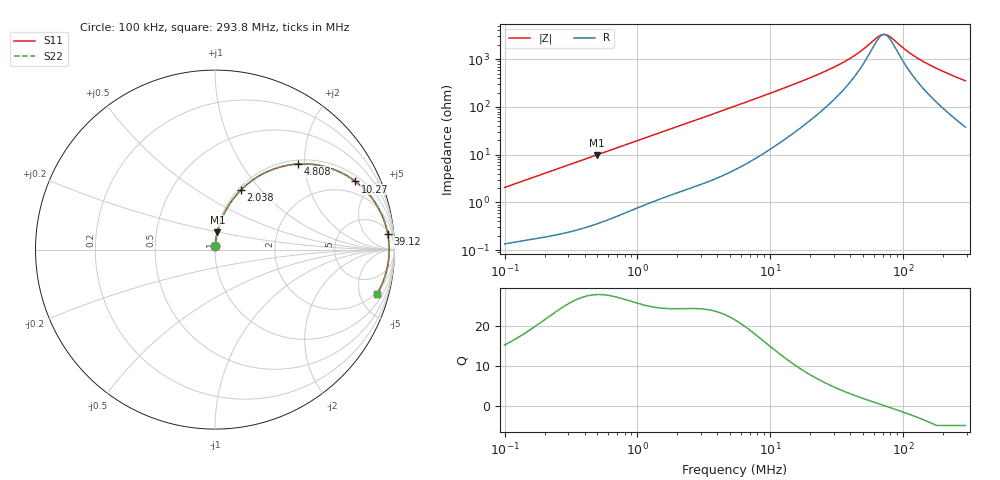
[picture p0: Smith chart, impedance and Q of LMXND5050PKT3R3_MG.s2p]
! LMXND5050PKT3R3_MG  S-PARAMETER MODEL  ( General Type )
! Model Generated by TAIYO YUDEN Corporation (http://www.ty-top.com)
! Version 1.0
! TAIYO YUDEN Control No. 191023NI43SB-FBB
! Copyright(c) 2019 TAIYO YUDEN CO.,LTD. All Rights Reserved.
! Product Description (link to TY-COMPAS)
! https://ds.yuden.co.jp/TYCOMPAS/or/detail?pn=LMXND5050PKT3R3NMG&u=M
! Products Name : Inductors
! Characteristics :
!  Inductance : 3.3 uH , SRF(min) : 48 MHz , DC Resistance(max) : 0.096 Ohm
!  Rated Current : Saturation :2350 mA , Temp Rise : 1700 mA
!  Case Size : 4.9 x 4.9 / 0.193 x 0.193 [mm/inch] , Thickness : 1.4 / 0.055 [mm/inch]
!  (Conditions: Temperature = 25 degC , DC Bias Current/Voltage = 0A / 0V)
! External Node Assignments :
!  1  o---GGG---o  2
! GND o---------o GND
! Frequency Range : 0.1MHz  -  293.796821MHz  [ 402 STEP ]
# MHz S RI R 50
! Freq[MHz].  S11 Real  S11 Imag  S21 Real  S21 Imag  S12 Real  S12 Imag  S22 Real  S22 Imag
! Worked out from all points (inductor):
!   401 points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, 100 kHz to 293.8 MHz, reference 50 ohm
!   read as one part in series: L = 3.24 uH near 104.1 kHz
!   highest Q = 27.9 at 493.9 kHz (marker M1), where L = 3.17 uH
!   self-resonance near 71.71 MHz
!   S11 on the Smith chart (normalised r, x): 100 kHz: 1.00, +0.04; 2.038 MHz: 1.03, +0.79; 4.808 MHz: 1.08, +1.84; 10.27 MHz: 1.27, +3.97; 39.12 MHz: 7, +19; 293.8 MHz: 1.75, -6.99
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0.1  0.00176 0.0204  0.9982 -0.0204  0.9982 -0.0204  0.00176 0.0204
0.380976  0.00851 0.0753  0.9915 -0.0753  0.9915 -0.0753  0.00851 0.0753
0.493866  0.013 0.0968  0.987 -0.0968  0.987 -0.0968  0.013 0.0968
1.451429  0.0831 0.2564  0.9169 -0.2564  0.9169 -0.2564  0.0831 0.2564
2.037923  0.1444 0.3316  0.8556 -0.3316  0.8556 -0.3316  0.1444 0.3316
3.038017  0.2624 0.4199  0.7376 -0.4199  0.7376 -0.4199  0.2624 0.4199
4.808425  0.4605 0.4767  0.5395 -0.4767  0.5395 -0.4767  0.4605 0.4767
5.420303  0.5178 0.477  0.4822 -0.477  0.4822 -0.477  0.5178 0.477
7.312659  0.6555 0.449  0.3445 -0.449  0.3445 -0.449  0.6555 0.449
10.26756  0.7825 0.3796  0.2175 -0.3796  0.2175 -0.3796  0.7825 0.3796
14.41648  0.8686 0.2947  0.1314 -0.2947  0.1314 -0.2947  0.8686 0.2947
20.65007  0.9222 0.2091  0.0778 -0.2091  0.0778 -0.2091  0.9222 0.2091
29.579  0.9506 0.1362  0.0494 -0.1362  0.0494 -0.1362  0.9506 0.1362
39.11697  0.9622 0.0883  0.0378 -0.0883  0.0378 -0.0883  0.9622 0.0883
48.72328  0.9673 0.0546  0.0327 -0.0546  0.0327 -0.0546  0.9673 0.0546
65.73373  0.9703 0.012  0.0297 -0.012  0.0297 -0.012  0.9703 0.012
71.19815  0.9705 0.000989  0.0295 -0.000989  0.0295 -0.000989  0.9705 0.000989
78.67184  0.9704 -0.0128  0.0296 0.0128  0.0296 0.0128  0.9704 -0.0128
108.2782  0.967 -0.0584  0.033 0.0584  0.033 0.0584  0.967 -0.0584
137.5887  0.961 -0.0957  0.039 0.0957  0.039 0.0957  0.961 -0.0957
197.081  0.9433 -0.1603  0.0567 0.1603  0.0567 0.1603  0.9433 -0.1603
293.7968  0.9025 -0.2478  0.0975 0.2478  0.0975 0.2478  0.9025 -0.2478
